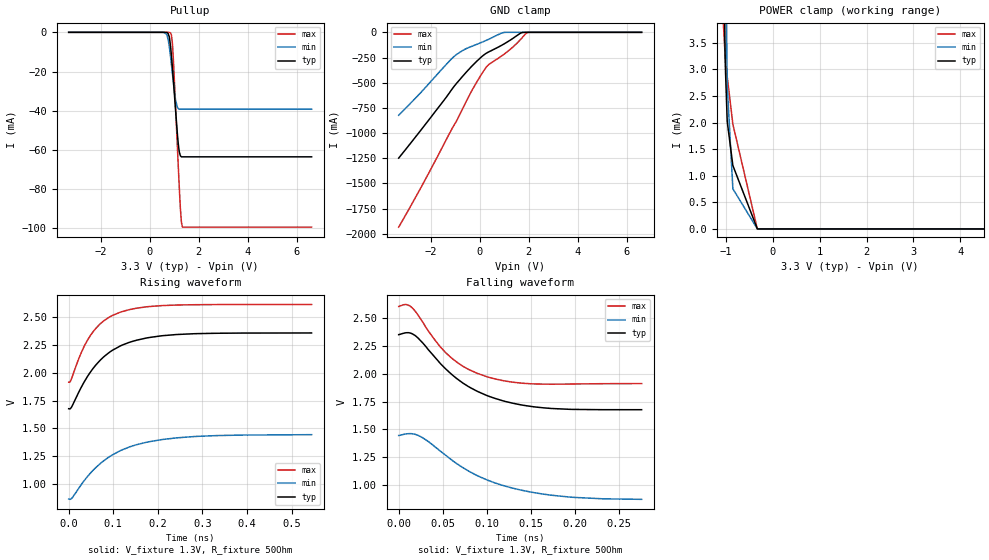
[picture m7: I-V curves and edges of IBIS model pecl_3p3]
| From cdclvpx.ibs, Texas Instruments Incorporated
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|   Pecl_3p3 Model   |
[Model]   pecl_3p3
Model_type   Open_source
Polarity   Non-Inverting
Vmeas = 2.09
Vref = 1.3
Cref = 1pF
Rref = 50
|   typ   min   max
|   (nom PVT)   (fast PVT)   (slow PVT)
C_comp   1.982e-13   1.121e-13   2.635e-13
[Model Spec]
|Subparameter
Vmeas   2.029V   1.174V   2.284V
| Vmeas is the expected cross point for each differential signal pair.
| Where nom  PVT is Nominal Process, 2.5V, 40C
|   Fast PVT is Strong Process,  2.625V, -40C
|   Slow PVT is Weak Process,   2.375V,100C
[Voltage Range]   3.3   2.375   3.6
|Junction Temperature
[Temperature range]   40   100   -40
[Pullup Reference]   3.3   2.375   3.6
[Pulldown Reference]   0   0   0
[Power Clamp Reference]   3.3   2.375   3.6
[GND Clamp Reference]   0   0   0
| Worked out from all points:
|   falling waveform, V_fixture 1.3V, R_fixture 50Ohm: 20-80 % time 64.4ps typ, 79.7ps min, 49.7ps max; typ from 2.35 V to 1.68 V
|   rising waveform, V_fixture 1.3V, R_fixture 50Ohm: 20-80 % time 85.8ps typ, 107ps min, 65.4ps max; typ from 1.68 V to 2.35 V
[GND Clamp]
|   Voltage   I(typ)   I(min)   I(max)
-3.3V     -1.248A    -823.2mA   -1.934A
-2.407V   -974.6mA   -600.7mA   -1.547A
-1.025V   -531.1mA   -236mA     -914.1mA
-712.8mV  -442mA     -183.6mA   -767.7mA
-330mV    -338.8mA   -139.8mA   -583.7mA
165mV     -225.5mA   -90.89mA   -381.7mA
408mV     -189.8mA   -64.14mA   -312.7mA
986.9mV   -116.2mA   -1.504mA   -218.4mA
1.391V    -54.13mA   -14.36nA   -138.2mA
1.672V    -8.174mA   0A         -69.97mA
1.924V    -4.082uA   0A         -4.711mA
6.6V      0A         0A         0A
[Pullup]
|   Voltage   I(typ)   I(min)   I(max)
-3.3V     0A         0A         0A
573.6mV   -1.198uA   -35.75uA   -722.5pA
751.8mV   -563.3uA   -3.538mA   -2.85uA
858mV     -7.823mA   -13.16mA   -406.2uA
924mV     -17.41mA   -20.66mA   -5.207mA
973.2mV   -25.54mA   -26.34mA   -15.3mA
1.056V    -39.65mA   -34.43mA   -37.72mA
1.168V    -56.97mA   -38.87mA   -68.59mA
1.251V    -62.97mA   -39.22mA   -89.49mA
1.294V    -63.53mA   -39.22mA   -96.88mA
1.337V    -63.53mA   -39.22mA   -99.38mA
6.6V      -63.53mA   -39.22mA   -99.41mA
[POWER Clamp]
|   Voltage   I(typ)   I(min)   I(max)
-3.3V     1.056A     1.064A     1.05A
-1.053V   6.043mA    12.47mA    3.832mA
-1.018V   3.291mA    6.608mA    3.281mA
-1.013V   3.084mA    6.053mA    3.233mA
-972.5mV  2.038mA    2.765mA    2.871mA
-970.8mV  2.013mA    2.682mA    2.857mA
-851.4mV  1.193mA    755.6uA    1.969mA
-330mV    1.901uA    1.178uA    1.883uA
6.6V      0A         0A         0A
[Ramp]
R_load = 50
|   typ   min   max
dV/dt_r   0.406093/8.53479e-11   0.345231/1.07186e-10   0.416507/6.53158e-11
dV/dt_f   0.406066/6.44397e-11   0.345221/8.00258e-11   0.416467/4.95151e-11
[Falling Waveform]
V_fixture = 1.3V
V_fixture_min = 0.375V
V_fixture_max = 1.6V
R_fixture = 50Ohm
|   Time   V(typ)   V(min)   V(max)
0s        2.354V     1.445V     2.608V
8.4ps     2.371V     1.46V      2.625V
18.4ps    2.347V     1.457V     2.569V
41.6ps    2.147V     1.341V     2.301V
57.8ps    2.013V     1.24V      2.159V
79.2ps    1.887V     1.127V     2.042V
100.2ps   1.806V     1.046V     1.975V
138.8ps   1.722V     954.5mV    1.918V
173.2ps   1.689V     908.4mV    1.908V
276.2ps   1.678V     870.8mV    1.913V
[Rising Waveform]
V_fixture = 1.3V
V_fixture_min = 0.375V
V_fixture_max = 1.6V
R_fixture = 50Ohm
|   Time   V(typ)   V(min)   V(max)
0s        1.677V     869.9mV    1.914V
6.6ps     1.692V     874.9mV    1.947V
22.8ps    1.826V     966.9mV    2.126V
33.8ps    1.909V     1.029V     2.226V
53.8ps    2.031V     1.123V     2.359V
79.2ps    2.142V     1.213V     2.463V
116.2ps   2.238V     1.302V     2.54V
172.8ps   2.307V     1.375V     2.586V
243.8ps   2.34V      1.417V     2.603V
545ps     2.353V     1.445V     2.608V
